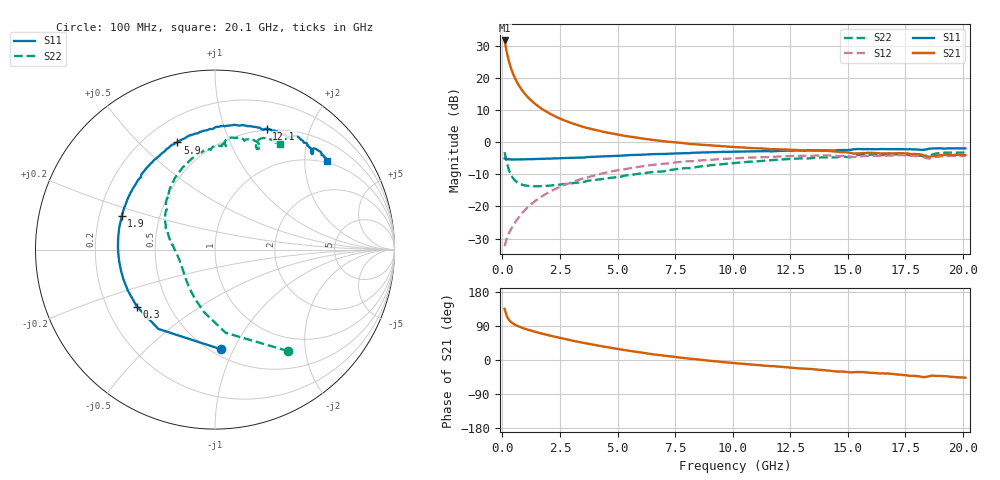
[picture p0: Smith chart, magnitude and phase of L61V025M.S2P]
!  Infineon Technologies AG
! BFR380L3 , PF131585-7, No.6, Th 09.10.01, soldered on pcb-board, measured with PP GSG850
!  Vce=1.0 V,  Ic=25.0 mA
! Common Emitter S-Parameters:  15. November 2001
#  GHz  S  MA  R  50
! f  S11  S21  S12  S22
! GHz  Mag  Ang  Mag  Ang  Mag  Ang  Mag  Ang
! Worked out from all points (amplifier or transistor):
!   201 points, 100 MHz to 20.1 GHz, reference 50 ohm
!   highest |S21| = 31.6 dB at 100 MHz (marker M1)
!   |S21| within 3 dB of that: start of sweep to 177 MHz
!   unconditionally stable (mu >= 1): 1.172 GHz to 4.824 GHz
!   at 3.4 GHz: K = 1.02, MAG = 7.4 dB, |S12| = -11.5 dB
!   at 10.1 GHz: K = 0.97, MSG = 1.7 dB, |S12| = -5.0 dB
!   at 20.1 GHz: K = 0.99, MSG = 0.1 dB, |S12| = -4.3 dB
!   S11 on the Smith chart (normalised r, x): 100 MHz: 0.56, -0.89; 300 MHz: 0.33, -0.29; 1.9 GHz: 0.30, +0.16; 5.9 GHz: 0.33, +0.66; 12.1 GHz: 0.49, +1.40; 20.1 GHz: 0.94, +2.57
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0.1  0.556 -86.7  38.01 134.9  0.02414 57.8  0.697 -54.2
0.2  0.543 -125.5  24.27 114.7  0.03242 52.7  0.4676 -82.6
0.3  0.5389 -143.9  17.26 105.1  0.03941 54.2  0.3556 -99.6
0.4  0.5365 -154.9  13.29 99.1  0.04586 56.6  0.2976 -111.8
0.5  0.5365 -162.0  10.77 94.9  0.05259 58.9  0.2645 -121.1
0.6  0.5368 -167.5  9.044 91.6  0.05988 60.7  0.2439 -128.6
0.7  0.5376 -172.0  7.801 88.8  0.06674 62.1  0.2307 -134.8
0.8  0.5383 -175.5  6.851 86.3  0.07421 63.2  0.2219 -139.9
1  0.5409 178.7  5.524 82.1  0.08919 64.3  0.2118 -148.0
1.2  0.543 173.7  4.63 78.3  0.1041 64.7  0.2076 -154.1
1.5  0.5475 167.4  3.74 73.2  0.1271 64.5  0.2058 -161.1
1.9  0.5529 160.3  2.992 66.9  0.1574 63.0  0.2086 -168.2
2.6  0.5636 149.1  2.242 57.0  0.2087 59.2  0.2204 -177.6
3.5  0.5777 136.4  1.729 45.4  0.2722 53.1  0.2379 173.1
4.6  0.6041 123.0  1.395 33.2  0.342 45.2  0.2752 161.9
5.9  0.6329 109.3  1.163 20.6  0.4127 35.9  0.3215 149.7
6.8  0.6529 100.7  1.053 12.9  0.4546 29.1  0.349 140.9
10.1  0.7109 76.8  0.8365 -8.2  0.5602 7.8  0.4741 115.4
12.1  0.7315 66.8  0.7683 -18.0  0.5994 -3.7  0.5363 100.8
13.5  0.7422 60.0  0.7382 -24.5  0.6145 -11.8  0.5672 91.8
16.8  0.777 48.1  0.6724 -36.0  0.6172 -26.8  0.642 73.2
20.1  0.7979 38.4  0.6304 -46.7  0.6103 -39.9  0.6912 58.4
